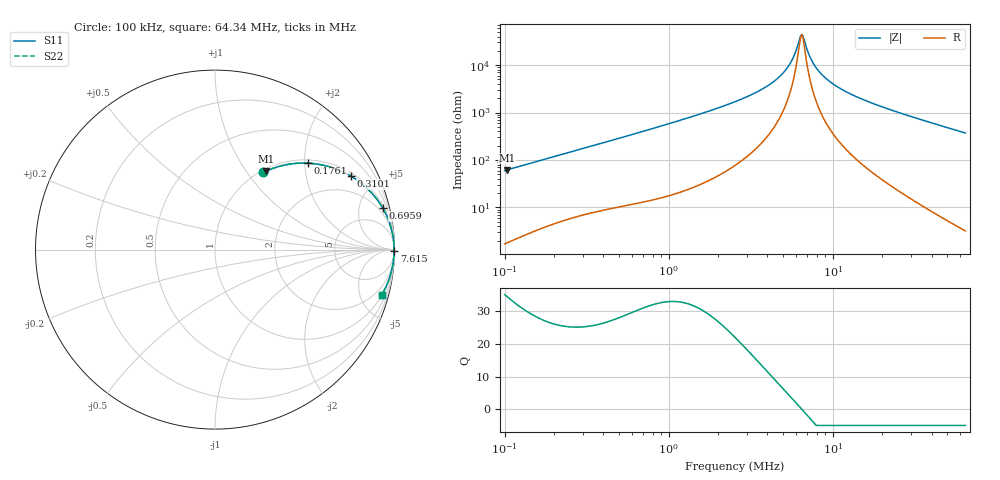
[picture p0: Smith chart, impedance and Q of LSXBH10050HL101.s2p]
! LSXBH10050HL101  S-PARAMETER MODEL  ( General Type )
! Model Generated by TAIYO YUDEN Corporation (http://www.ty-top.com)
! Version 3.0
! TAIYO YUDEN Control No. 180118NI43SB-FBB
! Copyright(c) 2007 TAIYO YUDEN CO.,LTD. All Rights Reserved.
! Product Description (link to TY-COMPAS)
! https://ds.yuden.co.jp/TYCOMPAS/or/detail?pn=LSXBH10050HL101M&u=M
! Products Name : Inductors
! Characteristics :
!  Inductance : 100 uH , SRF(min) : 4.6 MHz , DC Resistance(max) : 0.2717 Ohm
!  Rated Current : Saturation :1300 mA , Temp Rise : 1200 mA (40 degC)
!  Case Size : 10.0 x 9.8 / 0.394 x 0.386 [mm/inch] , Thickness : 5 / 0.197 [mm/inch]
!  (Conditions: Temperature = 25 degC , DC Bias Current/Voltage = 0A / 0V)
! External Node Assignments :
!  1  o---GGG---o  2
! GND o---------o GND
! Frequency Range : 0.1MHz  -  64.339822MHz  [ 402 STEP ]
# MHz S RI R 50
! Freq[MHz].  S11 Real  S11 Imag  S21 Real  S21 Imag  S12 Real  S12 Imag  S22 Real  S22 Imag
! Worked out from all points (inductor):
!   401 points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, 100 kHz to 64.34 MHz, reference 50 ohm
!   read as one part in series: L = 94.9 uH near 103.3 kHz
!   highest Q = 34.5 at 103.3 kHz (marker M1), where L = 95.3 uH
!   self-resonance near 6.375 MHz
!   S11 on the Smith chart (normalised r, x): 100 kHz: 1.03, +1.20; 176.1 kHz: 1.08, +2.08; 310.1 kHz: 1.14, +3.60; 695.9 kHz: 1.26, +8.00; 7.615 MHz: open; 64.34 MHz: 1.06, -7.41
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0.1  0.2701 0.43  0.7299 -0.43  0.7299 -0.43  0.2701 0.43
0.103286  0.2825 0.436  0.7175 -0.436  0.7175 -0.436  0.2825 0.436
0.176093  0.5199 0.4815  0.4801 -0.4815  0.4801 -0.4815  0.5199 0.4815
0.295407  0.7392 0.4197  0.2608 -0.4197  0.2608 -0.4197  0.7392 0.4197
0.310087  0.7562 0.4101  0.2438 -0.4101  0.2438 -0.4101  0.7562 0.4101
0.695895  0.9347 0.2315  0.0653 -0.2315  0.0653 -0.2315  0.9347 0.2315
0.872651  0.9567 0.1886  0.0433 -0.1886  0.0433 -0.1886  0.9567 0.1886
2.53653  0.9939 0.0586  0.00613 -0.0586  0.00613 -0.0586  0.9939 0.0586
3.678981  0.9965 0.0324  0.00347 -0.0324  0.00347 -0.0324  0.9965 0.0324
4.765042  0.9974 0.0169  0.00261 -0.0169  0.00261 -0.0169  0.9974 0.0169
5.511344  0.9976 0.00879  0.00237 -0.00879  0.00237 -0.00879  0.9976 0.00879
5.879526  0.9977 0.00524  0.0023 -0.00524  0.0023 -0.00524  0.9977 0.00524
6.272304  0.9977 0.0017  0.00227 -0.0017  0.00227 -0.0017  0.9977 0.0017
6.478426  0.9977 -6.06e-05  0.00226 6.06e-05  0.00226 6.06e-05  0.9977 -6.06e-05
6.691322  0.9977 -0.00182  0.00226 0.00182  0.00226 0.00182  0.9977 -0.00182
7.493079  0.9977 -0.00803  0.0023 0.00803  0.0023 0.00803  0.9977 -0.00803
7.615203  0.9977 -0.00892  0.00232 0.00892  0.00232 0.00892  0.9977 -0.00892
8.807898  0.9975 -0.0171  0.00252 0.0171  0.00252 0.0171  0.9975 -0.0171
10.86796  0.9969 -0.0295  0.00309 0.0295  0.00309 0.0295  0.9969 -0.0295
14.53883  0.9954 -0.049  0.00462 0.049  0.00462 0.049  0.9954 -0.049
22.13506  0.9906 -0.0847  0.00945 0.0847  0.00945 0.0847  0.9906 -0.0847
64.33982  0.9303 -0.2503  0.0697 0.2503  0.0697 0.2503  0.9303 -0.2503
